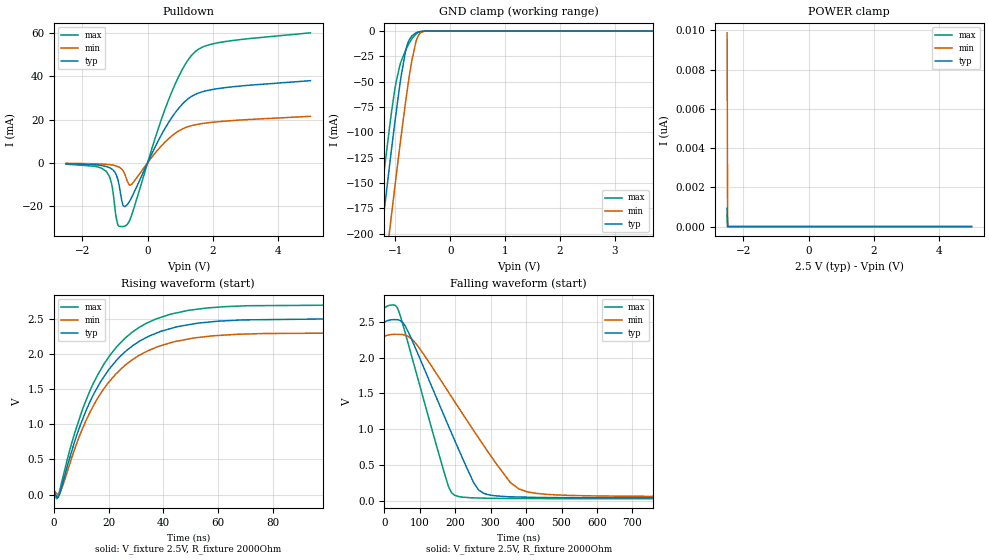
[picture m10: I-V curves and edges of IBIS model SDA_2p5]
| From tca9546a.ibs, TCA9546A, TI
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|   Model
[Model]   SDA_2p5
Model_type   I/O_open_drain
Polarity   Non-Inverting
Enable   Active-Low
Vinl = 0.75
Vinh = 1.75
Vmeas = 1.25
Vref = 2.5
Cref = 1pF
Rref = 2000
|   typ   min   max
C_comp   3.666pF   3.611pF   3.839pF
[Voltage Range]   2.5   2.3   2.7
[Temperature Range]   27   125   -40
[Pullup Reference]   2.5   2.3   2.7
[Pulldown Reference]   -0   -0   -0
[Power Clamp Reference]   2.5   2.3   2.7
[GND Clamp Reference]   -0   -0   -0
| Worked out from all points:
|   slope of the pulldown table from 0 to 0.375 V, typ, clamps not added: 32.4 ohm
|   GND clamp passes 1 mA (typ) near -0.59 V on its own axis
|   falling waveform, V_fixture 2.5V, R_fixture 2000Ohm: 20-80 % time 128ns typ, 180ns min, 90.2ns max; typ from 2.5 V to 0.037 V
|   rising waveform, V_fixture 2.5V, R_fixture 2000Ohm: 20-80 % time 19.5ns typ, 20ns min, 19.1ns max; typ from 0.037 V to 2.5 V
[Pulldown]
|   Voltage   I(typ)   I(min)   I(max)
-2.5V     -400.6uA   -210uA     -619.7uA
-1.262V   -1.718mA   -710.6uA   -4.029mA
-1.105V   -2.759mA   -978.6uA   -9.516mA
-917.5mV  -7.35mA    -1.685mA   -28.4mA
-767.5mV  -18.96mA   -3.363mA   -29.42mA
-700mV    -20.21mA   -5.167mA   -29.26mA
-520mV    -16.87mA   -10.26mA   -25.4mA
537.5mV   15.99mA    9.633mA    24.89mA
950mV     25.14mA    14.67mA    39.76mA
1.37V     30.89mA    17.25mA    50.01mA
2.21V     34.38mA    19.04mA    55.57mA
4.992V    37.93mA    21.48mA    60.02mA
[GND Clamp]
|   Voltage   I(typ)   I(min)   I(max)
-2.5V     -804.9mA   -869mA     -765mA
-1.323V   -233.1mA   -298.9mA   -192.4mA
-1.248V   -197.9mA   -263.6mA   -157.6mA
-1.09V    -125.7mA   -190.5mA   -88.23mA
-992.5mV  -83.17mA   -146.4mA   -52.1mA
-917.5mV  -52.95mA   -113.5mA   -33.8mA
-812.5mV  -19.58mA   -69.72mA   -18.9mA
-700mV    -4.935mA   -29.28mA   -7.673mA
-625mV    -1.839mA   -10.66mA   -2.994mA
-542.5mV  -471.1uA   -1.967mA   -678.6uA
-407.5mV  -26.82uA   -81.51uA   -28.19uA
4.992V    0A         0A         0A
[POWER Clamp]
|   Voltage   I(typ)   I(min)   I(max)
-2.5V     940.2pA    9.878nA    629.1pA
-2.485V   0A         0A         0A
-2.478V   0A         0A         0A
4.992V    0A         0A         0A
[Ramp]
R_load = 2000
|   typ   min   max
dV/dt_r   1.47762/1.94942e-08   1.34644/2.00012e-08   1.60427/1.91333e-08
dV/dt_f   1.47762/1.27568e-07   1.34644/1.80308e-07   1.60427/9.00955e-08
[Falling Waveform]
V_fixture = 2.5V
V_fixture_min = 2.3V
V_fixture_max = 2.7V
R_fixture = 2000Ohm
C_fixture = 0F
|   Time   V(typ)   V(min)   V(max)
0s        2.5V       2.3V       2.7V
28.5ns    2.53V      2.325V     2.733V
42.43ns   2.522V     2.325V     2.622V
85.09ns   2.162V     2.218V     1.875V
168.3ns   1.19V      1.613V     401.9mV
198ns     846.4mV    1.386V     75.23mV
266.4ns   145mV      872.3mV    35.79mV
354.8ns   53.15mV    255.8mV    29.24mV
403.9ns   46.92mV    121.4mV    28.31mV
1us       37.3mV     55.92mV    26.21mV
[Rising Waveform]
V_fixture = 2.5V
V_fixture_min = 2.3V
V_fixture_max = 2.7V
R_fixture = 2000Ohm
C_fixture = 0F
|   Time   V(typ)   V(min)   V(max)
0s        37.3mV     55.92mV    26.21mV
1.041ns   -32.12mV   14.32mV    -58.41mV
1.921ns   -13.2mV    14.8mV     24.67mV
7.704ns   767.2mV    657.3mV    888.1mV
13.23ns   1.324V     1.175V     1.482V
18.06ns   1.665V     1.496V     1.843V
23.14ns   1.923V     1.735V     2.112V
37.36ns   2.297V     2.097V     2.501V
62.36ns   2.473V     2.271V     2.675V
1us       2.5V       2.3V       2.7V
